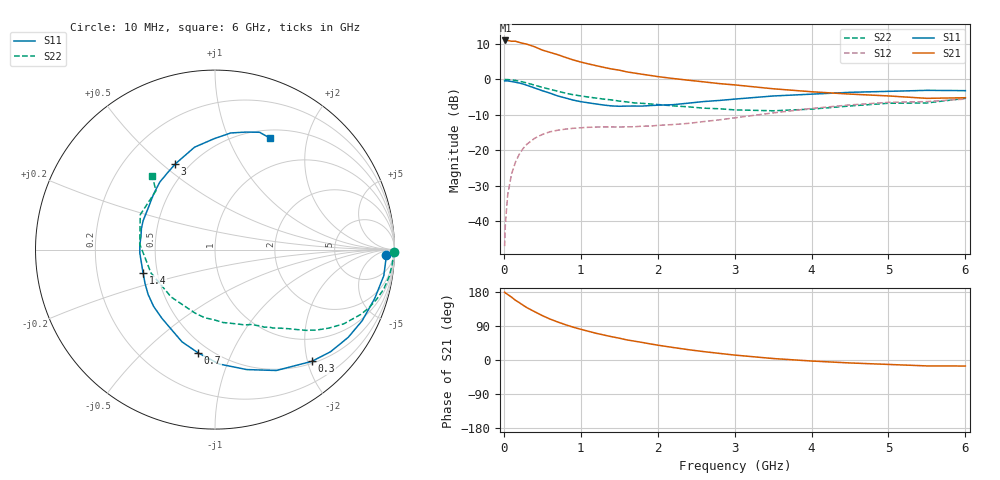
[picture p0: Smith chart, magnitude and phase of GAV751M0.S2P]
! Infineon Technologies  Discrete & RF Semiconductors
! BF775
! Si NPN RF Bipolar Junction Transistor in SOT23
! VCE = 0.75 V  IC = 1 mA
! Common Emitter S-Parameters:  May  1996
# GHz  S  MA  R  50
!  f  S11  S21  S12  S22
! GHz  MAG  ANG  MAG  ANG  MAG  ANG  MAG  ANG
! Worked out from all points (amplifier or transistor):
!   36 points, 10 MHz to 6 GHz, reference 50 ohm
!   highest |S21| = 11.0 dB at 20 MHz (marker M1)
!   |S21| within 3 dB of that: start of sweep to 543.3 MHz
!   unconditionally stable (mu >= 1): 1.33 GHz to end of sweep
!   at 250 MHz: K = 0.22, MSG = 14.9 dB, |S12| = -19.6 dB
!   at 1.4 GHz: K = 1.05, MAG = 6.9 dB, |S12| = -13.4 dB
!   at 6 GHz: K = 1.10, MAG = -1.7 dB, |S12| = -5.6 dB
!   S11 on the Smith chart (normalised r, x): 10 MHz: 30, -18; 300 MHz: 0.54, -2.08; 700 MHz: 0.43, -0.75; 1.4 GHz: 0.42, -0.13; 3 GHz: 0.42, +0.55; 6 GHz: 0.60, +1.43
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0.01  0.9517 -1.7  3.462 179.0  0.0044 88.4  0.9996 -0.8
0.02  0.9535 -3.6  3.543 177.0  0.009 89.7  0.9932 -1.8
0.05  0.9516 -8.8  3.543 172.9  0.0233 83.9  0.9911 -4.5
0.1  0.9306 -17.0  3.453 165.9  0.0459 79.3  0.9824 -8.7
0.15  0.9107 -25.8  3.459 157.8  0.0672 73.6  0.9653 -13.2
0.25  0.8592 -41.5  3.22 144.6  0.1053 63.9  0.9171 -20.7
0.3  0.8238 -49.1  3.138 138.1  0.1212 59.8  0.8888 -24.0
0.4  0.7553 -63.1  2.885 127.5  0.147 51.9  0.8277 -30.0
0.5  0.6913 -75.2  2.59 117.1  0.1664 45.8  0.7716 -34.5
0.6  0.638 -87.9  2.405 108.1  0.1817 40.6  0.7243 -38.2
0.7  0.5833 -99.2  2.231 100.3  0.1912 36.4  0.679 -41.5
0.9  0.5095 -117.9  1.882 86.7  0.2034 30.4  0.6063 -46.7
1.1  0.466 -137.2  1.652 75.7  0.2101 26.3  0.5621 -51.1
1.4  0.4215 -162.0  1.401 61.5  0.213 22.9  0.5121 -57.6
1.7  0.4197 176.4  1.226 49.7  0.214 24.0  0.4642 -63.8
2.2  0.4388 147.8  1.028 33.0  0.2298 26.6  0.4221 -77.0
3  0.5259 114.9  0.835 13.0  0.2858 29.4  0.3704 -107.7
3.5  0.5819 101.3  0.736 3.9  0.3357 27.3  0.3598 -132.7
4.5  0.6558 82.3  0.619 -7.8  0.4354 16.9  0.4206 175.8
5  0.6769 75.3  0.583 -11.7  0.4728 9.8  0.4596 154.9
5.5  0.6993 69.2  0.539 -15.6  0.4849 2.4  0.4642 135.1
6  0.6924 63.8  0.55 -15.9  0.5264 -1.6  0.5388 130.5
